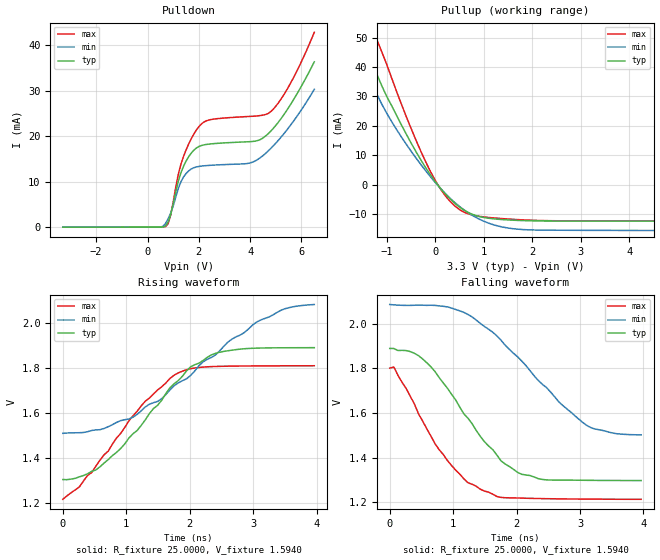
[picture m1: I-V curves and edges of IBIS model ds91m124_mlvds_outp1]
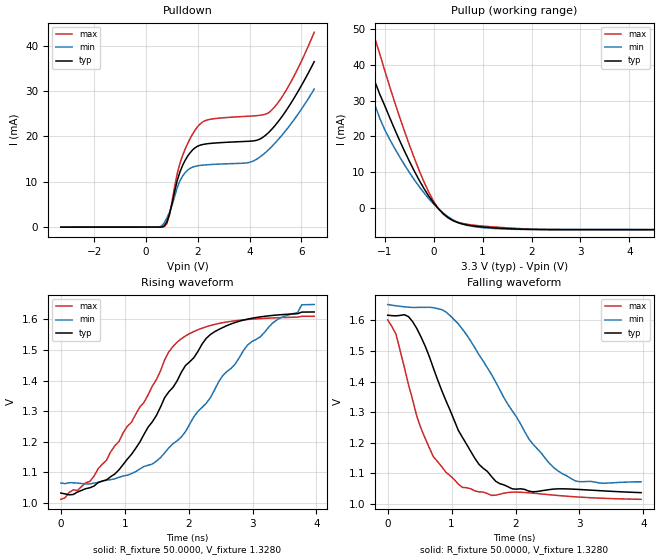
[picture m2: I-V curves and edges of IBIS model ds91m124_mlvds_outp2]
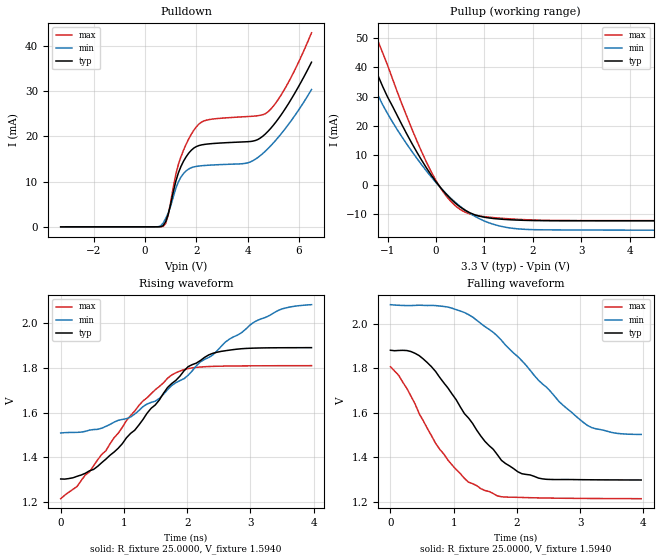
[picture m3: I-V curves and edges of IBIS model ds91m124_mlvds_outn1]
|   National Semiconductor Corporation
|   IBIS Model of DS91M124
[IBIS Ver]   3.2
[File name]   ds91m124.ibs
[File Rev]   1.0
[Date]   25/7/08
[Source]
[Notes]
Created by Shrikant G Kadadevar
[Disclaimer]
(C) Copyright National Semiconductor Corporation 2008
   All rights reserved
National Semiconductor Corporation hereby grants the
user of this IBIS model a non-exclusive, nontransferable
license to use this IBIS model under the following terms.
Before using this IBIS model, the user should read this
license.  If the user does not accept these terms,  the
IBIS model should be returned to National within 30 days.
The user is granted this license only to use the
IBIS model and is not granted rights to sell, load, rent,
lease or license the IBIS model in whole or in part, or in
modified form to anyone other than user. User may modify
the IBIS model to suit its specific applications but rights
to derivative works and such modifications shall belong to
National.
This IBIS model is provided on an "AS IS" basis and
National makes absolutely no warranty with respect to the
information contained herein.NATIONAL DISCLAIMS AND CUSTOMER
WAIVES ALL WARRANTIES, EXPRESS OR IMPLIED, INCLUDING
WARRANTIES OF MERCHANTABILITY OR FITNESS FOR A PARTICULAR
PURPOSE. The entire risk as to quality and performance is
with the Customer. ACCORDINGLY, IN NO EVENT SHALL THE
COMPANY BE LIABLE FOR ANY DAMAGES, WHETHER IN CONTRACT OR
TORT,INCLUDING ANY LOST PROFITS OR OTHER INCIDENTAL,
CONSEQUENTIAL, EXEMPLARY, OR PUNITIVE DAMAGES ARISING OUT
OF THE USE OR APPLICATION OF THE IBIS model provided in
this package.Further, National reserves the right to make
changes without notice to any product herein to improve
reliability, function, or design. National does not convey
any license under patent rights or any other intellectual
property rights, including those of third parties.
National is not obligated to provide maintenance or support
for the licensed IBIS model.
[Copyright]  Copyright 2008, National Semiconductor, All Rights Reserved
[Component]  DS91M124
Si_location Pin
Timing_location Pin
[Manufacturer]  National Semiconductor Corp
[Package]
|   typ   min   max
R_pkg   0   0   0
L_pkg   0   0   0
C_pkg   0   0   0
[Pin]   signal_name   model_name   R_pin   L_pin   C_pin
1   DE0   ds91m124_cmos_in1
2   DE1   ds91m124_cmos_in1
3   DE2   ds91m124_cmos_in1
4   VDD   POWER
5   GND   GND
6   DI   ds91m124_cmos_in4
7   NC   NC
8   DE3   ds91m124_cmos_in1
9   B3   ds91m124_mlvds_outn
10   A3   ds91m124_mlvds_outp
11   A2   ds91m124_mlvds_outp
12   B2   ds91m124_mlvds_outn
13   B1   ds91m124_mlvds_outn
14   A1   ds91m124_mlvds_outp
15   A0   ds91m124_mlvds_outp
16   B0   ds91m124_mlvds_outn
[Diff pin]  inv_pin  vdiff  tdelay_typ  tdelay_min  tdelay_max
10 9   0   0.0s   0.0s   0.0s
11 12  0   0.0s   0.0s   0.0s
14 13  0   0.0s   0.0s   0.0s
15 16  0   0.0s   0.0s   0.0s
|Electrical package information. Will overide all the default values.
[Package Model] SOIC_16
[Model Selector]   ds91m124_mlvds_outp
ds91m124_mlvds_outp1   Use this model for 50-ohm loads
ds91m124_mlvds_outp2   Use this model for 100-ohm loads
[Model Selector]   ds91m124_mlvds_outn
ds91m124_mlvds_outn1   Use this model for 50-ohm loads
ds91m124_mlvds_outn2   Use this model for 100-ohm loads
[Define Package Model]  SOIC_16
[Manufacturer]   National Semiconductor
[Description]   16 SOIC, DS91M124
[OEM]   NA
[Number Of Pins]   16
[Pin Numbers]
   1   |   1 = 01
   2   |   2 = 02
   3   |   3 = 03
   4   |   4 = 04
   5   |   5 = 05
   6   |   6 = 06
   7   |   7 = 07
   8   |   8 = 08
   9   |   9 = 09
  10   |  10 = 10
  11   |  11 = 11
  12   |  12 = 12
  13   |  13 = 13
  14   |  14 = 14
  15   |  15 = 15
  16   |  16 = 16
[Model Data]
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[End Model Data]
[End Package Model]
| Models and submodels in the file (6): ds91m124_mlvds_outp1 (Output), ds91m124_mlvds_outp2 (Output), ds91m124_mlvds_outn1 (Output), ds91m124_mlvds_outn2 (Output), ds91m124_cmos_in1 (Input), ds91m124_cmos_in4 (Input)
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|   Model ds91m124_mlvds_outp1
[Model]  ds91m124_mlvds_outp1
Model_type Output
Polarity   Non-Inverting
Vmeas =  1.56V
Rref =   25.0000
Vref =   1.56V
C_comp   7.359p   6.991p  7.743p
[Temperature Range]   25.0000   85.0000   -40.0000
[Voltage Range]   3.3000V   3.0000V   3.6000V
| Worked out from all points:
|   slope of the pullup table from 0 to 0.495 V, typ, clamps not added: 57.8 ohm
|   rising waveform, R_fixture 25.0000, V_fixture 1.5940: 20-80 % time 1.08ns typ, 1.61ns min, 1ns max; typ from 1.3 V to 1.89 V
|   falling waveform, R_fixture 25.0000, V_fixture 1.5940: 20-80 % time 928ps typ, 1.2ns min, 780ps max; typ from 1.89 V to 1.3 V
[Pulldown]
|Voltage   I(typ)   I(min)   I(max)
-3.3V     -16.04uA   -15.04uA   -17.07uA
500mV     -2.06uA    10.82uA    -4.562uA
700mV     234.6uA    784.7uA    91.14uA
900mV     2.713mA    3.039mA    2.586mA
1.2V      10.09mA    8.499mA    11.63mA
1.4V      13.34mA    10.98mA    15.49mA
2V        17.72mA    13.33mA    22.08mA
2.5V      18.31mA    13.61mA    23.68mA
4V        18.79mA    14.11mA    24.35mA
4.8V      21.08mA    17.27mA    25.39mA
5.6V      27.19mA    22.62mA    31.92mA
6.5V      36.35mA    30.31mA    42.84mA
[Pullup]
|Voltage   I(typ)   I(min)   I(max)
-3.3V     175.7mA    142.4mA    190.6mA
-1.7V     63.82mA    53.26mA    77.6mA
-1.5V     51.44mA    43.29mA    64.96mA
-1.3V     41.45mA    34.36mA    54.06mA
-800mV    23.56mA    18.75mA    31.69mA
-400mV    11.23mA    9.085mA    15.15mA
-100mV    3.299mA    2.667mA    4.432mA
200mV     -3.058mA   -2.926mA   -3.666mA
600mV     -8.75mA    -8.684mA   -9.419mA
1.2V      -11.61mA   -13.63mA   -11.3mA
1.8V      -12.2mA    -15.25mA   -11.96mA
6.5V      -12.39mA   -15.63mA   -12.32mA
[Ramp]
| variable   typ   min   max
dV/dt_r  0.3567/1.100n   0.3514/1.640n   0.3599/1.010n
dV/dt_f  0.3578/0.936n   0.3457/1.180n   0.3610/0.798n
R_load = 25.00
[Rising Waveform]
R_fixture= 25.0000
V_fixture= 1.5940
V_fixture_min= 1.7950
V_fixture_max= 1.5120
|time   V(typ)   V(min)   V(max)
0s        1.303V     1.509V     1.215V
260ps     1.315V     1.512V     1.27V
585ps     1.36V      1.526V     1.389V
1.3ns     1.569V     1.627V     1.652V
1.82ns    1.745V     1.734V     1.779V
2.015ns   1.806V     1.768V     1.798V
2.47ns    1.871V     1.876V     1.808V
3.12ns    1.89V      2.015V     1.81V
3.51ns    1.891V     2.066V     1.81V
3.965ns   1.891V     2.084V     1.811V
[Falling Waveform]
R_fixture= 25.0000
V_fixture= 1.5940
V_fixture_min= 1.7950
V_fixture_max= 1.5120
|time   V(typ)   V(min)   V(max)
0s        1.889V     2.086V     1.801V
65ps      1.889V     2.084V     1.806V
585ps     1.825V     2.082V     1.529V
975ps     1.684V     2.07V      1.365V
1.43ns    1.495V     2.001V     1.259V
1.755ns   1.386V     1.926V     1.223V
2.08ns    1.326V     1.833V     1.219V
2.665ns   1.3V       1.651V     1.216V
3.12ns    1.299V     1.542V     1.215V
3.965ns   1.298V     1.502V     1.214V
|   Model ds91m124_mlvds_outp2
[Model] ds91m124_mlvds_outp2
Model_type Output
Polarity   Non-Inverting
Vmeas =  1.56V
Rref =   50.0000
Vref =   1.56V
C_comp   7.359p   6.991p  7.743p
[Temperature Range]   25.0000   85.0000   -40.0000
[Voltage Range]   3.3000V   3.0000V   3.6000V
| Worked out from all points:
|   slope of the pullup table from 0 to 0.495 V, typ, clamps not added: 89.8 ohm
|   rising waveform, R_fixture 50.0000, V_fixture 1.3280: 20-80 % time 1.1ns typ, 1.33ns min, 1.01ns max; typ from 1.03 V to 1.62 V
|   falling waveform, R_fixture 50.0000, V_fixture 1.3280: 20-80 % time 738ps typ, 1.02ns min, 589ps max; typ from 1.62 V to 1.04 V
[Pulldown]
|Voltage   I(typ)   I(min)   I(max)
-3.3V     -16.03uA   -15.03uA   -17.07uA
500mV     -1.779uA   19.11uA    -4.505uA
700mV     266.1uA    947.9uA    95.95uA
900mV     2.789mA    3.225mA    2.636mA
1.2V      10.22mA    8.651mA    11.74mA
1.4V      13.49mA    11.17mA    15.63mA
2V        17.87mA    13.53mA    22.22mA
2.5V      18.47mA    13.8mA     23.81mA
4V        18.95mA    14.28mA    24.48mA
4.8V      21.23mA    17.43mA    25.52mA
5.6V      27.34mA    22.77mA    32.05mA
6.5V      36.5mA     30.45mA    42.97mA
[Pullup]
|Voltage   I(typ)   I(min)   I(max)
-3.3V     175.6mA    142.3mA    190.5mA
-1.7V     63.38mA    52.81mA    76.23mA
-1.6V     56.8mA     47.64mA    68.59mA
-1.5V     50.5mA     42.58mA    62.09mA
-1.3V     39.51mA    33.04mA    51.53mA
-1.2V     35.24mA    28.74mA    47.34mA
-900mV    25.28mA    19.17mA    33.99mA
-200mV    5.404mA    4.186mA    7.28mA
100mV     -330.9uA   -343uA     -296.8uA
500mV     -4.222mA   -4.121mA   -4.112mA
1.6V      -5.915mA   -6.038mA   -5.727mA
6.5V      -6.152mA   -6.146mA   -6.187mA
[Ramp]
| variable   typ   min   max
dV/dt_r  0.3571/1.190n   0.3519/1.440n   0.3593/1.070n
dV/dt_f  0.3557/0.812n   0.3514/1.110n   0.3588/0.645n
R_load = 50.00
[Rising Waveform]
R_fixture= 50.0000
V_fixture= 1.3280
V_fixture_min= 1.3569
V_fixture_max= 1.3117
|time   V(typ)   V(min)   V(max)
0s        1.032V     1.065V     1.011V
455ps     1.049V     1.062V     1.07V
845ps     1.094V     1.078V     1.186V
1.43ns    1.264V     1.127V     1.381V
1.69ns    1.363V     1.18V      1.494V
1.885ns   1.427V     1.215V     1.537V
2.275ns   1.538V     1.325V     1.576V
2.6ns     1.58V      1.43V      1.592V
3.315ns   1.613V     1.589V     1.605V
3.965ns   1.625V     1.649V     1.61V
[Falling Waveform]
R_fixture= 50.0000
V_fixture= 1.3280
V_fixture_min= 1.3569
V_fixture_max= 1.3117
|time   V(typ)   V(min)   V(max)
0s        1.617V     1.652V     1.601V
130ps     1.615V     1.647V     1.554V
325ps     1.612V     1.643V     1.39V
650ps     1.482V     1.643V     1.184V
1.17ns    1.218V     1.571V     1.054V
1.755ns   1.066V     1.373V     1.032V
2.21ns    1.042V     1.212V     1.037V
2.6ns     1.049V     1.119V     1.029V
2.99ns    1.047V     1.073V     1.023V
3.965ns   1.037V     1.072V     1.015V
|   Model ds91m124_mlvds_outn1
[Model]  ds91m124_mlvds_outn1
Model_type Output
Polarity   Inverting
Vmeas =  1.56V
Rref =   25.0000
Vref =   1.56V
C_comp   7.359p   6.991p  7.743p
[Temperature Range]   25.0000   85.0000   -40.0000
[Voltage Range]   3.3000V   3.0000V   3.6000V
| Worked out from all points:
|   slope of the pullup table from 0 to 0.495 V, typ, clamps not added: 57.8 ohm
|   rising waveform, R_fixture 25.0000, V_fixture 1.5940: 20-80 % time 1.08ns typ, 1.61ns min, 1ns max; typ from 1.3 V to 1.89 V
|   falling waveform, R_fixture 25.0000, V_fixture 1.5940: 20-80 % time 916ps typ, 1.2ns min, 785ps max; typ from 1.88 V to 1.3 V
[Pulldown]
|Voltage   I(typ)   I(min)   I(max)
-3.3V     -16.04uA   -15.04uA   -17.07uA
500mV     -2.06uA    10.82uA    -4.562uA
700mV     234.6uA    784.7uA    91.14uA
900mV     2.713mA    3.039mA    2.586mA
1.2V      10.09mA    8.499mA    11.63mA
1.4V      13.34mA    10.98mA    15.49mA
2V        17.72mA    13.33mA    22.08mA
2.5V      18.31mA    13.61mA    23.68mA
4V        18.79mA    14.11mA    24.35mA
4.8V      21.08mA    17.27mA    25.39mA
5.6V      27.19mA    22.62mA    31.92mA
6.5V      36.35mA    30.31mA    42.84mA
[Pullup]
|Voltage   I(typ)   I(min)   I(max)
-3.3V     175.7mA    142.4mA    190.6mA
-1.7V     63.82mA    53.26mA    77.6mA
-1.5V     51.44mA    43.29mA    64.96mA
-1.3V     41.45mA    34.36mA    54.06mA
-800mV    23.56mA    18.75mA    31.69mA
-400mV    11.23mA    9.085mA    15.15mA
-100mV    3.299mA    2.667mA    4.432mA
200mV     -3.058mA   -2.926mA   -3.666mA
600mV     -8.75mA    -8.684mA   -9.419mA
1.2V      -11.61mA   -13.63mA   -11.3mA
1.8V      -12.2mA    -15.25mA   -11.96mA
6.5V      -12.39mA   -15.63mA   -12.32mA
[Ramp]
| variable   typ   min   max
dV/dt_r  0.3567/1.100n   0.3514/1.640n   0.3599/1.010n
dV/dt_f  0.3578/0.936n   0.3457/1.180n   0.3610/0.798n
R_load = 25.00
[Rising Waveform]
R_fixture= 25.0000
V_fixture= 1.5940
V_fixture_min= 1.7950
V_fixture_max= 1.5120
|time   V(typ)   V(min)   V(max)
0s        1.303V     1.509V     1.215V
260ps     1.315V     1.512V     1.27V
585ps     1.36V      1.526V     1.389V
1.3ns     1.569V     1.627V     1.652V
1.82ns    1.745V     1.734V     1.779V
2.015ns   1.806V     1.768V     1.798V
2.47ns    1.871V     1.876V     1.808V
3.12ns    1.89V      2.015V     1.81V
3.51ns    1.891V     2.066V     1.81V
3.965ns   1.891V     2.084V     1.811V
[Falling Waveform]
R_fixture= 25.0000
V_fixture= 1.5940
V_fixture_min= 1.7950
V_fixture_max= 1.5120
|time   V(typ)   V(min)   V(max)
0s        1.881V     2.086V     1.807V
260ps     1.88V      2.082V     1.71V
585ps     1.825V     2.082V     1.529V
975ps     1.684V     2.07V      1.365V
1.43ns    1.495V     2.001V     1.259V
1.755ns   1.386V     1.926V     1.223V
2.08ns    1.326V     1.833V     1.219V
2.665ns   1.3V       1.651V     1.216V
3.12ns    1.299V     1.542V     1.215V
3.965ns   1.298V     1.502V     1.214V
